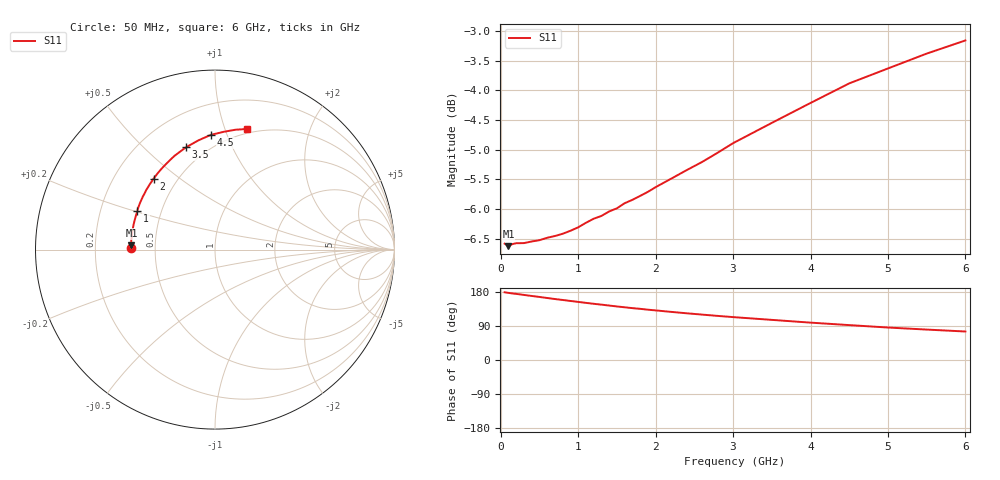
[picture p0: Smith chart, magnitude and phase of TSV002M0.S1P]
! SIEMENS Small Signal Semiconductors
! BAT14-03W
! Si Schottky Diode in SOD323
! IF = 2 mA
! S-Parameters:  November  1995
# GHz  S  MA  R  50
!  f  S11
! GHz  MAG  ANG
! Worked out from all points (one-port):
!   34 points, 50 MHz to 6 GHz, reference 50 ohm
!   lowest |S11| = -6.6 dB at 100 MHz (marker M1), VSWR 2.75, Z = 18.2 + j1.1 ohm
!   |S11| at or under -10 dB: nowhere
!   S11 on the Smith chart (normalised r, x): 50 MHz: 0.36, +0.01; 1 GHz: 0.36, +0.21; 2 GHz: 0.37, +0.40; 3.5 GHz: 0.39, +0.68; 4.5 GHz: 0.41, +0.88; 6 GHz: 0.46, +1.19
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0.05  0.4688 178.7
0.1  0.4665 177.1
0.15  0.4683 175.7
0.2  0.4692 174.5
0.4  0.4707 169.0
0.5  0.4719 166.4
0.6  0.4741 163.6
0.8  0.4778 158.4
1  0.4838 153.3
1.2  0.4919 148.3
1.3  0.4946 146.1
1.4  0.4989 143.7
1.5  0.502 141.3
1.6  0.507 139.1
1.7  0.5103 136.9
1.8  0.5142 135.0
1.9  0.5182 132.8
2  0.523 130.9
2.2  0.5316 127.0
2.4  0.5405 123.3
2.8  0.559 116.4
3  0.5696 113.2
3.5  0.5924 105.9
4  0.6157 98.6
4.5  0.6395 92.1
5  0.6583 85.7
5.5  0.6775 80.3
6  0.695 75.2
